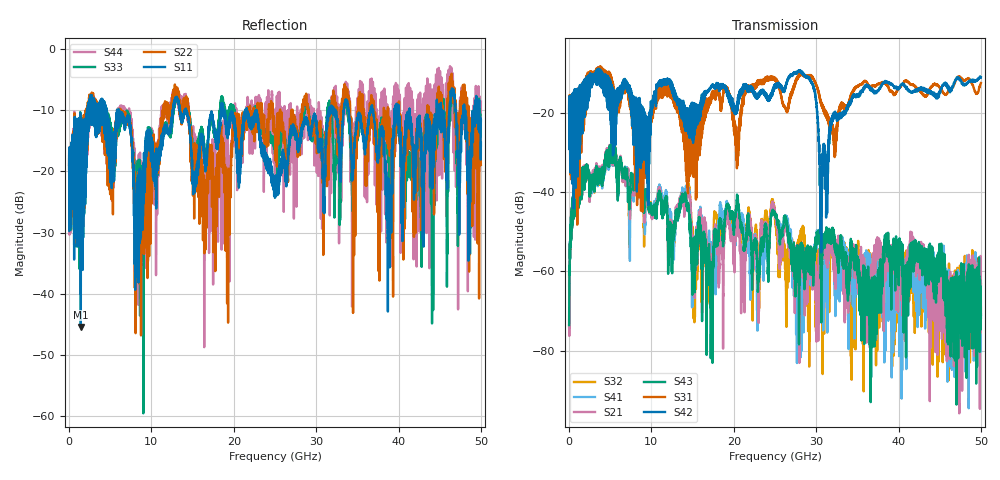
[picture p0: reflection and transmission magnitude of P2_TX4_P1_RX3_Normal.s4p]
!Keysight Technologies,N5225B,MY57041031,A.13.20.10
!Date: Friday, May 31, 2019 11:18:13
!Correction: S11(Full 4 Port(1,2,3,4))
!S12(Full 4 Port(1,2,3,4))
!S13(Full 4 Port(1,2,3,4))
!S14(Full 4 Port(1,2,3,4))
!S21(Full 4 Port(1,2,3,4))
!S22(Full 4 Port(1,2,3,4))
!S23(Full 4 Port(1,2,3,4))
!S24(Full 4 Port(1,2,3,4))
!S31(Full 4 Port(1,2,3,4))
!S32(Full 4 Port(1,2,3,4))
!S33(Full 4 Port(1,2,3,4))
!S34(Full 4 Port(1,2,3,4))
!S41(Full 4 Port(1,2,3,4))
!S42(Full 4 Port(1,2,3,4))
!S43(Full 4 Port(1,2,3,4))
!S44(Full 4 Port(1,2,3,4))
!S4P File: Measurements: <S11,S12,S13,S14>,
!<S21,S22,S23,S24>,
!<S31,S32,S33,S34>,
!<S41,S42,S43,S44>:
# Hz S  dB  R 50.0
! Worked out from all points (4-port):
!   5000 points, 10 MHz to 50 GHz, reference 50 ohm
!   strongest paths, dB at 10 MHz, 12.51 GHz, 25.01 GHz, 37.51 GHz, 50 GHz:
!     S42: -19.7, -14.4, -13.1, -14.4, -11.1
!     S31: -19.3, -14.1, -11.3, -12.8, -12.5
!     S43: -73.5, -55.0, -45.6, -59.9, -71.6
!     S21: -74.0, -51.5, -45.8, -52.8, -70.8
!     S41: -63.1, -53.6, -45.4, -60.1, -71.2
!     S32: -60.5, -53.1, -47.0, -68.1, -63.2
!   lowest |S11| = -45.4 dB at 1.43 GHz (marker M1), VSWR 1.01, Z = 49.5 + j0.112 ohm
!   |S11| at or under -10 dB: 6.023 GHz to 12.61 GHz (6.592 GHz wide, 70.7 % of centre); 14.2 GHz to 18.43 GHz (4.229 GHz wide, 25.9 % of centre); 22.71 GHz to 31.52 GHz (8.807 GHz wide, 32.5 % of centre)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
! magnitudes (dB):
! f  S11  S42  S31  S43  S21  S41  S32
! 10 MHz  -18.9  -19.7  -19.3  -73.5  -74.0  -63.1  -60.5
! 1.43 GHz  -45.4  -20.0  -26.8  -39.4  -39.0  -39.1  -38.9
! 17.19 GHz  -10.9  -13.7  -17.3  -63.7  -56.6  -52.8  -59.4
! 24.82 GHz  -21.7  -13.7  -11.0  -45.2  -43.5  -44.7  -44.0
! 28.02 GHz  -15.9  -9.3  -10.3  -58.8  -61.7  -66.9  -54.1
! 30.63 GHz  -14.7  -40.9  -17.8  -61.3  -57.3  -54.7  -66.0
! 50 GHz  -15.3  -11.1  -12.5  -71.6  -70.8  -71.2  -63.2
